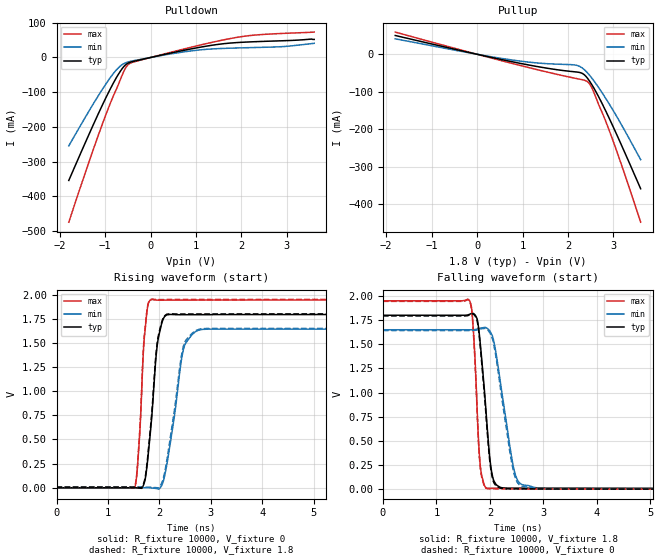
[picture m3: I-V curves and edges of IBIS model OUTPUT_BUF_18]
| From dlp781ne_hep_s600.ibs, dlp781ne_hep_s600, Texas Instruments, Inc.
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[Model]   OUTPUT_BUF_18
Model_type  Output
Vref =   0
Rref =   10000
Cref =   10p
Vmeas =   1.2
| variable   typ   min   max
C_comp   0.65pF   0.45pF   1.15pF
| C_pullup   0.66pF   0.45pF   1.15pF
| C_pulldown   0.63pF   0.50pF   1.03pF
[Temperature Range]   25   85   -40
[Voltage range]   1.8   1.65   1.95
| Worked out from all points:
|   slope of the pulldown table from 0 to 0.27 V, typ, clamps not added: 34.3 ohm
|   slope of the pullup table from 0 to 0.27 V, typ, clamps not added: 37.6 ohm
|   rising waveform, R_fixture 10000, V_fixture 0: 20-80 % time 164ps typ, 253ps min, 111ps max; typ from 0 V to 1.79 V
|   falling waveform, R_fixture 10000, V_fixture 1.8: 20-80 % time 159ps typ, 266ps min, 98.4ps max; typ from 1.8 V to 0.006 V
|   rising waveform, R_fixture 10000, V_fixture 1.8: 20-80 % time 164ps typ, 256ps min, 110ps max; typ from 0.006 V to 1.8 V
|   falling waveform, R_fixture 10000, V_fixture 0: 20-80 % time 159ps typ, 263ps min, 98.5ps max; typ from 1.79 V to 0 V
[Pulldown]
| OUTPUT_BUF_18
|   Voltage   I(typ)   I(min)   I(max)
-1.8V     -354.2mA   -254.4mA   -474.4mA
-1.265V   -195mA     -134.5mA   -266.6mA
-895mV    -92.67mA   -59.47mA   -134.6mA
-755mV    -58.61mA   -36.11mA   -91.94mA
-645mV    -35.65mA   -22.4mA    -56.96mA
-555mV    -21.67mA   -15.53mA   -31.37mA
-480mV    -15.3mA    -12.24mA   -19.11mA
-345mV    -10.18mA   -8.457mA   -11.8mA
875mV     24.33mA    18.74mA    29.04mA
1.865V    42.67mA    27.28mA    57.21mA
2.905V    48.22mA    31.33mA    69.32mA
3.6V      52.02mA    40.86mA    73.18mA
[Pullup]
| OUTPUT_BUF_18
|   Voltage   I(typ)   I(min)   I(max)
-1.8V     49.99mA    41.08mA    59.07mA
730mV     -18.9mA    -14.55mA   -23.06mA
1.36V     -33.47mA   -23.55mA   -42.08mA
2.165V    -46.93mA   -28.87mA   -64.13mA
2.32V     -51.32mA   -37.02mA   -67.96mA
2.435V    -64.68mA   -50.22mA   -73.6mA
2.49V     -74.19mA   -58.09mA   -81.45mA
2.545V    -84.87mA   -66.63mA   -94.28mA
2.7V      -119.1mA   -93.19mA   -140.9mA
2.895V    -167.2mA   -129.8mA   -198.5mA
3.195V    -246.7mA   -191.5mA   -300.4mA
3.6V      -358.2mA   -280.8mA   -447.3mA
[Ramp]
| OUTPUT_BUF_18
| variable   typ   min   max
dV/dt_r   1.08/1.67E-10   0.99/2.58E-10   1.17/1.11E-10
dV/dt_f   1.09/1.62E-10   1.00/2.72E-10   1.18/1.01E-10
R_load = 10000
[Rising Waveform]
| OUTPUT_BUF_18
R_fixture =   10000
C_fixture =   0
L_fixture =   0
V_fixture =   0
V_fixture_min = 0
V_fixture_max = 0
|   Time   V(typ)   V(min)   V(max)
0s        2.935nV    32.33nV    304.2pV
1.525ns   12.81uV    20.21uV    4.084mV
1.615ns   -3.833mV   105uV      533.5mV
1.71ns    58.13mV    123.1uV    1.568V
1.855ns   750.8mV    -2.782mV   1.947V
1.955ns   1.458V     -9.919mV   1.942V
2.08ns    1.753V     73.73mV    1.941V
2.47ns    1.791V     1.436V     1.942V
2.825ns   1.792V     1.638V     1.943V
24.99ns   1.793V     1.642V     1.944V
[Falling Waveform]
| OUTPUT_BUF_18
R_fixture =   10000
C_fixture =   0
L_fixture =   0
V_fixture =   1.8
V_fixture_min = 1.65
V_fixture_max = 1.95
|   Time   V(typ)   V(min)   V(max)
0s        1.8V       1.65V      1.95V
1.62ns    1.81V      1.65V      1.949V
1.69ns    1.819V     1.651V     1.653V
1.76ns    1.764V     1.656V     844.3mV
1.82ns    1.507V     1.667V     244.5mV
1.955ns   601.1mV    1.662V     9.6mV
2.08ns    79.45mV    1.512V     9.328mV
2.475ns   9.39mV     152mV      8.293mV
2.885ns   8.404mV    13.17mV    7.567mV
24.99ns   6.04mV     6.675mV    5.66mV
[Rising Waveform]
| OUTPUT_BUF_18
R_fixture =   10000
C_fixture =   0
L_fixture =   0
V_fixture =   1.8
V_fixture_min = 1.65
V_fixture_max = 1.95
|   Time   V(typ)   V(min)   V(max)
0s        6.039mV    6.675mV    5.66mV
1.525ns   6.058mV    6.695mV    10.55mV
1.61ns    2.738mV    6.771mV    514.5mV
1.71ns    72.65mV    6.795mV    1.588V
1.855ns   789.8mV    4.171mV    1.952V
1.955ns   1.486V     187.2uV    1.948V
2.08ns    1.761V     104.7mV    1.948V
2.465ns   1.798V     1.459V     1.948V
2.825ns   1.798V     1.646V     1.949V
24.99ns   1.8V       1.65V      1.95V
[Falling Waveform]
| OUTPUT_BUF_18
R_fixture =   10000
C_fixture =   0
L_fixture =   0
V_fixture =   0
V_fixture_min = 0
V_fixture_max = 0
|   Time   V(typ)   V(min)   V(max)
0s        1.793V     1.642V     1.944V
1.62ns    1.803V     1.642V     1.942V
1.69ns    1.811V     1.643V     1.63V
1.76ns    1.748V     1.648V     814.7mV
1.815ns   1.504V     1.657V     253.2mV
1.955ns   560.3mV    1.649V     4.112mV
2.075ns   66.14mV    1.49V      3.651mV
2.465ns   3.348mV    135.5mV    2.653mV
2.86ns    2.404mV    7.718mV    1.943mV
24.99ns   6.498nV    37.43nV    3.212nV
